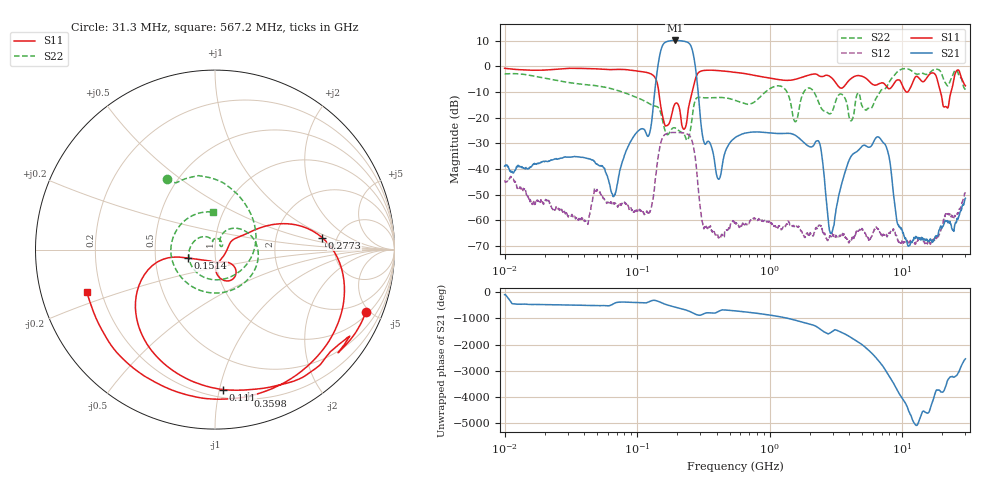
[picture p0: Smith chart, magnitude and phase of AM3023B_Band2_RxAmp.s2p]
# Hz S DB R 50.0
!freq dBS11 angS11 dBS21 angS21 dBS12 angS12 dBS22 angS22
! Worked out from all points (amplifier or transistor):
!   1601 points, 10 MHz to 30 GHz, reference 50 ohm
!   highest |S21| = 10.0 dB at 192.5 MHz (marker M1)
!   |S21| within 3 dB of that: 152.8 MHz to 258.4 MHz (105.7 MHz wide, 51.4 % of centre)
!   unconditionally stable (mu >= 1): start of sweep to end of sweep
!   at 37.85 MHz: K = 4029.69, MAG = -27.0 dB, |S12| = -59.6 dB
!   at 547.7 MHz: K = 5565.54, MAG = -23.9 dB, |S12| = -60.9 dB
!   at 30 GHz: K = 38854.80, MAG = -50.1 dB, |S12| = -49.1 dB
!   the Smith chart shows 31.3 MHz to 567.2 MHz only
!   S11 on the Smith chart (normalised r, x): 31.3 MHz: 1.18, -4.78; 111 MHz: 0.26, -1.03; 151.4 MHz: 0.74, -0.07; 277.3 MHz: 3.84, +0.80; 359.8 MHz: 0.22, -1.23; 567.2 MHz: 0.15, -0.16
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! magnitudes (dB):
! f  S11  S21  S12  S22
! 10 MHz  -0.8  -38.9  -44.4  -3.0
! 31.3 MHz  -0.8  -35.4  -58.7  -6.4
! 38.04 MHz  -0.9  -35.5  -59.2  -7.0
! 66.63 MHz  -1.3  -50.7  -53.2  -9.0
! 111 MHz  -2.1  -24.4  -57.0  -13.3
! 125.2 MHz  -2.8  -25.4  -56.8  -14.7
! 144.7 MHz  -8.9  1.4  -34.7  -16.2
! 151.4 MHz  -16.1  6.4  -29.5  -18.5
! 192.5 MHz  -14.8  10.0  -25.8  -24.0
! 228.2 MHz  -24.4  9.7  -26.1  -26.8
! 277.3 MHz  -4.4  -1.7  -37.4  -12.8
! 359.8 MHz  -1.5  -30.7  -63.2  -12.3
! 413.9 MHz  -1.7  -44.1  -66.5  -12.2
! 547.7 MHz  -2.4  -27.8  -60.9  -13.3
! 567.2 MHz  -2.5  -27.3  -61.6  -13.6
! 2.084 GHz  -3.1  -31.4  -66.2  -9.0
! 2.409 GHz  -3.9  -30.9  -62.1  -15.6
! 2.913 GHz  -4.4  -65.0  -66.5  -18.2
! 4.177 GHz  -4.6  -34.6  -67.3  -21.0
! 7.926 GHz  -8.8  -34.8  -64.9  -6.5
! 11.14 GHz  -9.8  -70.1  -68.5  -1.1
! 30 GHz  -7.6  -51.4  -49.1  -9.3
